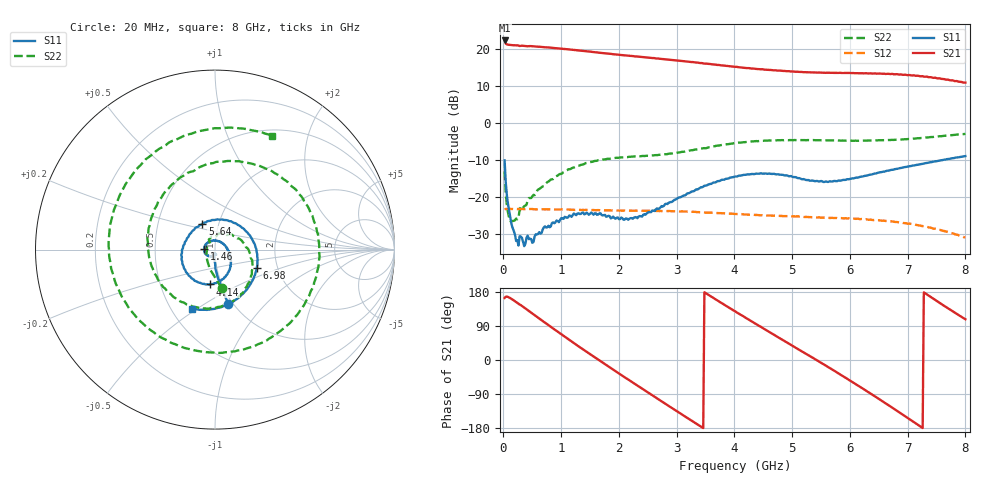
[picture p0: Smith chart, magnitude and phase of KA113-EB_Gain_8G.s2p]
!Agilent	"Technologies,E8364B,MY43040668,A.07.50.67"
!Agilent	E8364B:	A.07.50.67
!Date:	"Friday,"	February	"16,"	2018	10:35:35
!Correction:	S11(Full	2	"Port(1,2))"
!S21(Full	2	"Port(1,2))"
!S12(Full	2	"Port(1,2))"
!S22(Full	2	"Port(1,2))"
!S2P	File:	Measurements:	"S11,"	"S21,"	"S12,"	S22:
#	Hz	S	dB	R	50
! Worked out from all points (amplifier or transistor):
!   400 points, 20 MHz to 8 GHz, reference 50 ohm
!   highest |S21| = 22.3 dB at 20 MHz (marker M1)
!   |S21| within 3 dB of that: start of sweep to 1.488 GHz
!   unconditionally stable (mu >= 1): 50.91 MHz to end of sweep
!   at 1.34 GHz: K = 1.06, MAG = 20.0 dB, |S12| = -23.6 dB
!   at 4.02 GHz: K = 1.29, MAG = 16.7 dB, |S12| = -24.7 dB
!   at 8 GHz: K = 2.33, MAG = 14.5 dB, |S12| = -31.0 dB
!   S11 on the Smith chart (normalised r, x): 20 MHz: 0.95, -0.63; 1.46 GHz: 0.89, +0.01; 4.14 GHz: 0.88, -0.35; 5.64 GHz: 0.84, +0.25; 6.98 GHz: 1.56, -0.33; 8 GHz: 0.63, -0.48
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2e7  -10.17 -76.4  22.31 163.7  -23.44 17.2  -13.16 -79.9
8e7  -22.15 -89.4  21.15 166.3  -23.29 -1.7  -24.37 -143.0
4.8e8  -31.48 -99.3  20.78 124.9  -23.32 -36.8  -20.36 61.1
7.6e8  -28.30 -114.6  20.44 94.2  -23.43 -58.8  -16.05 18.1
1.06e9  -25.45 -141.4  19.99 61.8  -23.49 -82.0  -13.17 -18.8
1.36e9  -24.38 -172.3  19.50 29.9  -23.60 -105.3  -11.32 -50.1
1.46e9  -24.58 174.4  19.34 19.6  -23.57 -113.1  -10.83 -59.9
1.78e9  -25.44 133.3  18.80 -13.3  -23.69 -137.4  -9.82 -88.4
2.12e9  -25.87 81.9  18.25 -47.8  -23.75 -163.7  -9.30 -119.0
2.68e9  -23.28 0.2  17.43 -103.2  -23.85 152.8  -8.69 -171.1
3.06e9  -20.19 -28.9  16.84 -140.6  -24.01 122.9  -7.99 150.2
3.36e9  -18.06 -47.0  16.32 -170.0  -24.18 99.2  -7.16 119.6
4.02e9  -14.53 -90.2  15.15 127.8  -24.67 48.1  -5.49 59.1
4.14e9  -14.16 -98.1  14.94 116.5  -24.75 38.9  -5.26 49.2
4.62e9  -13.79 -137.0  14.34 72.6  -25.07 2.5  -4.78 11.2
5.34e9  -15.63 151.9  13.63 7.3  -25.57 -52.8  -4.67 -42.9
5.64e9  -15.89 116.0  13.55 -20.1  -25.74 -75.9  -4.73 -67.0
6.2e9  -14.56 48.9  13.44 -73.3  -26.04 -120.5  -4.83 -117.0
6.68e9  -12.90 3.1  13.25 -120.6  -26.63 -160.0  -4.68 -165.1
6.98e9  -11.92 -23.2  12.96 -150.9  -27.23 174.6  -4.44 163.0
7.4e9  -10.67 -59.7  12.36 166.4  -28.40 139.5  -3.85 119.1
8e9  -9.00 -111.6  10.90 107.6  -30.99 93.7  -2.99 63.1
